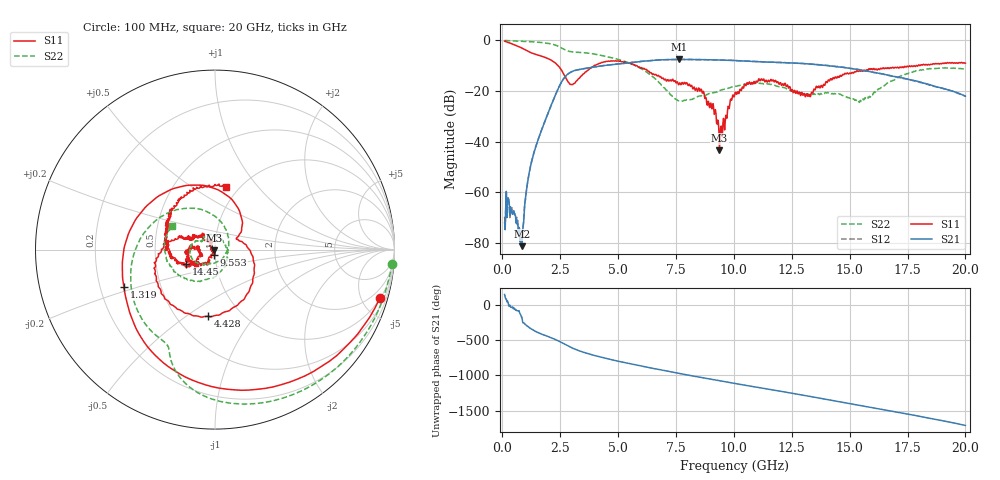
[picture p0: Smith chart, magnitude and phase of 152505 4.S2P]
!  2-Port S-parameters saved by WinCal
! VAR MeasName=S-Parameters (CALIBRATED_DATA) read from VNA (N5230C)
! VAR MeasDate=4/10/2015 9:28:49 AM
! VAR NAME=152505 4
! VAR FILENAME=152505 4.S2P
! VAR DATE=4/10/2015 9:28:49 AM
! VAR PHYS_PORTS=1,2
# Hz S DB R 50
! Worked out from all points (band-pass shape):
!   801 points, 100 MHz to 20 GHz, reference 50 ohm
!   highest |S21| = -7.54 dB at 7.637 GHz (marker M1); lowest = -81.2 dB at 846.2 MHz (marker M2)
!   |S21| within 3 dB of the highest: 3.99 GHz to 14.57 GHz (10.58 GHz wide, 114 % of centre)
!   lowest |S11| = -43.5 dB at 9.378 GHz (marker M3), VSWR 1.01, Z = 49.4 - j0.371 ohm
!   |S11| at or under -10 dB: 2.405 GHz to 3.97 GHz (1.565 GHz wide, 49.1 % of centre); 5.801 GHz to 17.88 GHz (12.08 GHz wide, 102 % of centre); 17.89819 GHz to 17.96076 GHz (62.58 MHz wide, 0.349 % of centre)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
!   |S22| runs from -24.5 to -0.1 dB; largest |S21 - S12| = 0.0066
!   S11 on the Smith chart (normalised r, x): 100 MHz: 1.03, -6.80; 1.319 GHz: 0.30, -0.18; 4.428 GHz: 0.70, -0.61; 9.553 GHz: 0.99, -0.06; 14.45 GHz: 0.71, -0.12; 20 GHz: 0.87, +0.69
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1e8  -0.37 -16.4  -71.94 147.6  -69.60 98.6  -0.08 -4.6
2.74125e8  -0.92 -41.0  -62.57 -2.3  -62.37 -1.5  -0.17 -11.5
8.4625e8  -3.06 -111.5  -81.18 -170.5  -81.02 175.5  -0.38 -34.3
1.070125e9  -4.13 -135.0  -57.44 63.7  -57.47 62.9  -0.48 -43.3
1.318875e9  -5.21 -157.5  -45.93 6.6  -45.86 6.8  -0.62 -53.5
2.164625e9  -8.15 114.1  -24.38 -112.1  -24.40 -112.0  -1.58 -91.0
2.93575e9  -17.43 27.4  -12.69 122.5  -12.68 122.7  -4.48 -116.2
3.43325e9  -13.95 -5.0  -11.37 57.1  -11.35 57.4  -4.81 -128.9
4.42825e9  -8.55 -96.2  -9.94 -33.9  -9.92 -33.7  -6.28 -165.1
5.497875e9  -8.98 -163.1  -8.87 -111.8  -8.82 -112.0  -9.02 149.1
6.741625e9  -13.85 159.1  -7.81 165.7  -7.79 165.4  -16.36 74.9
7.637125e9  -17.22 150.6  -7.54 108.6  -7.59 108.6  -23.96 -19.6
8.60725e9  -19.66 134.2  -7.65 50.5  -7.63 50.1  -21.85 -104.5
9.378375e9  -43.45 -146.1  -7.78 5.4  -7.81 5.4  -19.89 -126.0
9.5525e9  -30.82 -103.5  -7.85 -4.8  -7.86 -4.7  -19.37 -130.0
1.005e10  -20.83 -121.1  -7.99 -33.5  -8.00 -33.5  -18.22 -141.7
1.136838e10  -15.98 -166.9  -8.59 -107.5  -8.52 -107.3  -17.28 176.6
1.338325e10  -20.71 -153.6  -9.45 137.7  -9.40 137.8  -21.19 146.0
1.445288e10  -14.92 -153.8  -10.40 74.8  -10.38 74.7  -20.91 110.0
1.5423e10  -11.93 -170.5  -11.62 16.8  -11.61 15.8  -24.52 26.5
1.669162e10  -11.10 167.1  -13.81 -58.2  -13.91 -59.5  -16.50 -88.4
2e10  -9.04 79.9  -22.06 91.6  -22.09 92.2  -11.31 151.2
